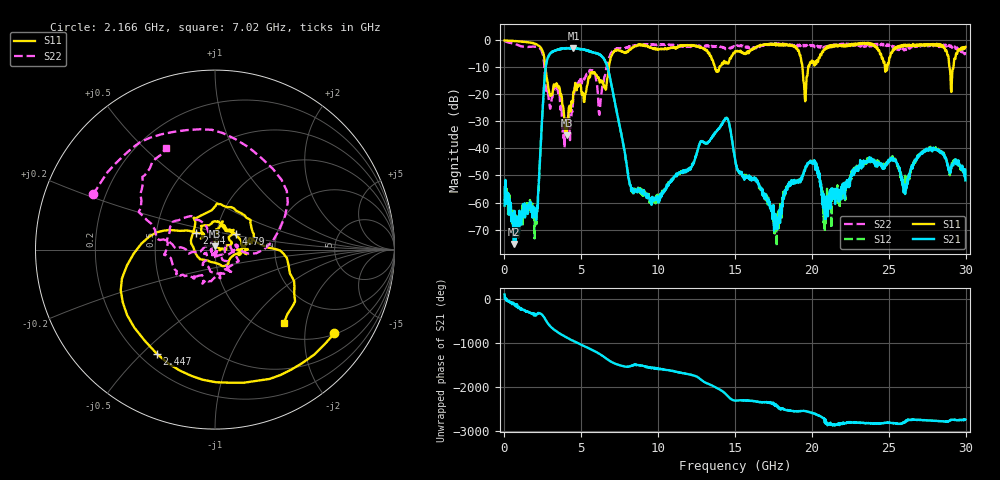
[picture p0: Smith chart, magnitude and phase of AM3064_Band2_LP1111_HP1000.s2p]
# Hz S DB R 50.0
!freq dBS11 angS11 dBS21 angS21 dBS12 angS12 dBS22 angS22
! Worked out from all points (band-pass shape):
!   1600 points, 10 MHz to 29.98 GHz, reference 50 ohm
!   highest |S21| = -2.80 dB at 4.49 GHz (marker M1); lowest = -75.3 dB at 609.8 MHz (marker M2)
!   |S21| within 3 dB of the highest: 2.868 GHz to 6.312 GHz (3.444 GHz wide, 75 % of centre)
!   lowest |S11| = -35.1 dB at 4.04 GHz (marker M3), VSWR 1.04, Z = 49.7 + j1.72 ohm
!   |S11| at or under -10 dB: 2.665 GHz to 6.785 GHz (4.121 GHz wide, 87.2 % of centre); 13.7 GHz to 13.98 GHz (282.2 MHz wide, 2.04 % of centre); 19.39 GHz to 19.75 GHz (369.2 MHz wide, 1.89 % of centre)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
!   |S22| runs from -39.9 to -0.1 dB; largest |S21 - S12| = 0.025
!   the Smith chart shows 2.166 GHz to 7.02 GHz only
!   S11 on the Smith chart (normalised r, x): 2.166 GHz: 1.03, -2.83; 2.447 GHz: 0.27, -0.55; 2.84 GHz: 0.80, +0.15; 4.79 GHz: 1.25, +0.22; 7.02 GHz: 1.25, -1.50
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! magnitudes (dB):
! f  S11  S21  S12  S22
! 10 MHz  0.0  -61.2  -53.9  -0.1
! 609.8 MHz  -0.2  -75.3  -65.6  -1.2
! 2.166 GHz  -1.8  -62.0  -62.1  -2.6
! 2.447 GHz  -3.6  -29.2  -29.2  -4.4
! 2.84 GHz  -17.1  -6.2  -6.1  -19.7
! 4.04 GHz  -35.1  -2.9  -2.8  -30.6
! 4.49 GHz  -19.0  -2.8  -2.9  -20.3
! 4.79 GHz  -16.7  -3.1  -3.1  -16.4
! 5.015 GHz  -19.3  -3.2  -3.2  -15.5
! 6.214 GHz  -15.5  -5.4  -5.3  -25.1
! 7.02 GHz  -5.0  -18.2  -18.0  -4.0
! 8.276 GHz  -2.7  -55.4  -55.1  -2.1
! 10 GHz  -3.3  -57.8  -57.9  -1.6
! 14.39 GHz  -8.5  -28.9  -28.9  -3.1
! 15 GHz  -4.0  -44.2  -44.0  -2.1
! 17.63 GHz  -1.8  -64.3  -64.8  -1.1
! 19.02 GHz  -2.8  -52.5  -52.3  -2.0
! 19.56 GHz  -22.5  -47.7  -47.5  -1.7
! 19.99 GHz  -7.5  -45.0  -45.1  -1.8
! 20.95 GHz  -2.9  -57.6  -63.7  -2.2
! 25 GHz  -8.4  -44.4  -44.9  -1.5
! 29.98 GHz  -2.4  -51.8  -49.5  -4.4
